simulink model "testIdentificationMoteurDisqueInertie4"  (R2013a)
settings: Solver=ode45  StartTime=0  StopTime=1  FixedStep=1e-3  MaxStep=SimParam2.Te  RelTol=1e-4  AbsTol=1e-4
PreLoadFcn:
  | warning('off','sm:sli:setup:compile:LocalSolverNotSupported')
model workspace (MAT data in the model file):
  handle : class17 (value not decoded)
  handle : class17 (value not decoded)
undefined symbols (not defined in the file or in its folder): SimParam2

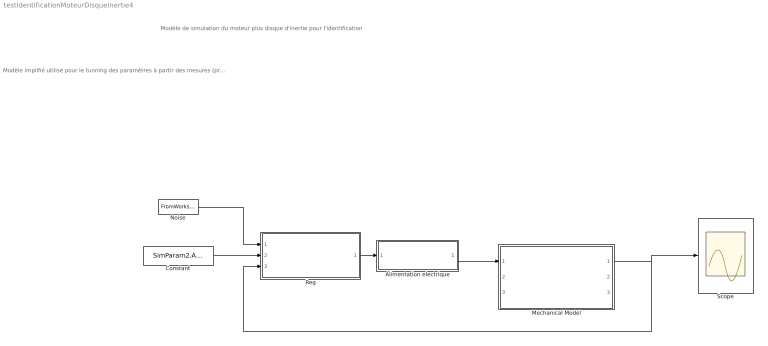
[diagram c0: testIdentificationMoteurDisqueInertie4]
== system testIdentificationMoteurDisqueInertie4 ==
  note: Modèle de simulation du moteur plus disque d'inertie pour l'identification
  note: Modèle implifié utilisé pour le tunning des paramètres à partir des mesures (prbs) effectuée sur le robot (Idem testIdentificationMoteur mais avec un élèment flexible dans le moteur) - Régulateur PID simple avec quantification codeur - Alimentation éléctrique modélisée par une fonction de transfert d'ordre deux avec delais (delais du contrôle) - Méchanique comprennant uniquement un modèle du moteur (inertie + frottement + 1ddl flexible en torsion) + frottement sec - Signaux d'exitation comprennant un bruit blanc et un signal cyclique (PRBS)
  Alimentation electrique : Subsystem
  Constant : Constant  Value=SimParam2.Alpha_c
  Mechanical Model : ModelReference  ModelNameDialog=MotorOnly_sm2.slx  SimulationMode=Normal  ModelReferenceVersion=1.261  CopyOfModelName=MotorOnly_sm2.slx  DefaultDataLogging=on
  Noise : FromWorkspace  VariableName=SimIn  SampleTime=SimParam2.Te  Interpolate=off  OutputAfterFinalValue=Holding final value
  Reg : Subsystem
  Scope : Scope
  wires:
  Noise/1 -> Reg/1(Noise)
  Reg/1(Torque) -> Alimentation electrique/1(Torque_in)
  Constant/1 -> Reg/2(Alpha_c)
  Alimentation electrique/1(Torque_out) -> Mechanical Model/1
  Mechanical Model/1 -> Reg/3(Alpha), Scope/1

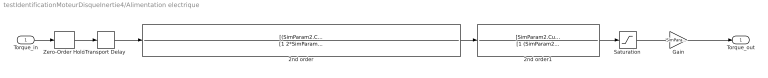
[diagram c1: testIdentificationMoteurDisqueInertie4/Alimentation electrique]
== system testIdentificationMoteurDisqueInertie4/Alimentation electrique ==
  Torque_in : Inport
  2nd order : TransferFcn  Numerator=[(SimParam2.CurrentLoop.f0*2*pi)^2]  Denominator=[1 2*SimParam2.CurrentLoop.Cr*(SimParam2.CurrentLoop.f0*2*pi) (SimParam2.CurrentLoop.f0*2*pi)^2]
  2nd order1 : TransferFcn  Numerator=[SimParam2.CurrentLoop.f1*2*pi]  Denominator=[1 (SimParam2.CurrentLoop.f1*2*pi)]
  Gain : Gain  Gain=SimParam2.Grel
  Saturation : Saturate  UpperLimit=10  LowerLimit=-10
  Transport Delay : TransportDelay  DelayTime=SimParam2.tauElec
  Zero-Order Hold : ZeroOrderHold  SampleTime=SimParam2.TeElec
  Torque_out : Outport
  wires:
  Saturation/1 -> Gain/1
  Torque_in/1 -> Zero-Order Hold/1
  Zero-Order Hold/1 -> Transport Delay/1
  2nd order/1 -> 2nd order1/1
  2nd order1/1 -> Saturation/1
  Gain/1 -> Torque_out/1
  Transport Delay/1 -> 2nd order/1

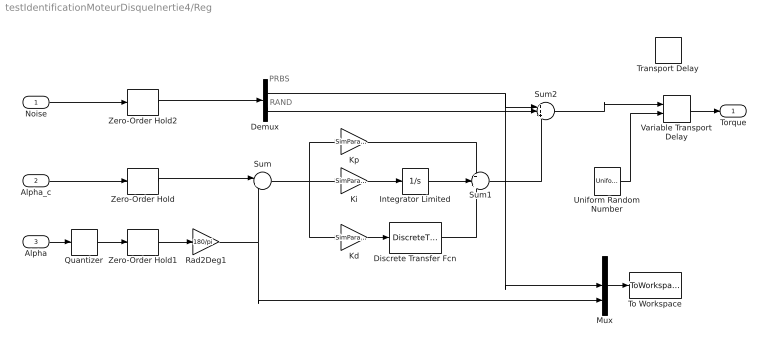
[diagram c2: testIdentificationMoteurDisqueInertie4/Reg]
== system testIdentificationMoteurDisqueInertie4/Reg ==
  note: RAND
  note: PRBS
  Noise : Inport
  Alpha_c : Inport  Port=2
  Alpha : Inport  Port=3
  Demux : Demux  Outputs=2
  Discrete Transfer Fcn : DiscreteTransferFcn  Numerator=[1 0 -1]  Denominator=[2 0 0]
  Integrator Limited : Integrator  LimitOutput=on  UpperSaturationLimit=1  LowerSaturationLimit=-1
  Kd : Gain  Gain=SimParam2.Control.Kd/SimParam2.Te
  Ki : Gain  Gain=SimParam2.Control.Ki*SimParam2.Te
  Kp : Gain  Gain=SimParam2.Control.Kp
  Mux : Mux  Inputs=3
  Quantizer : Quantizer  QuantizationInterval=SimParam2.CoderResol
  Rad2Deg1 : Gain  Gain=180/pi
  Sum : Sum  Inputs=|+-
  Sum1 : Sum  Inputs=+++
  Sum2 : Sum  Inputs=+++
  To Workspace : ToWorkspace  VariableName=simout  SampleTime=SimParam2.Te  SaveFormat=Structure With Time
  Transport Delay : TransportDelay  Commented=on  DelayTime=SimParam2.tauCtr
  Uniform Random Number : UniformRandomNumber  Minimum=SimParam2.tauCtr*0.9  Maximum=SimParam2.tauCtr*1.1  SampleTime=SimParam2.Te
  Variable Transport Delay : VariableTransportDelay  VariableDelayType=Variable transport delay  MaximumDelay=SimParam2.tauCtr*1.2
  Zero-Order Hold : ZeroOrderHold  SampleTime=SimParam2.Te
  Zero-Order Hold1 : ZeroOrderHold  SampleTime=SimParam2.Te
  Zero-Order Hold2 : ZeroOrderHold  SampleTime=SimParam2.Te
  Torque : Outport
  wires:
  Alpha_c/1 -> Zero-Order Hold/1
  Kd/1 -> Discrete Transfer Fcn/1
  Mux/1 -> To Workspace/1
  Zero-Order Hold/1 -> Sum/1
  Alpha/1 -> Quantizer/1
  Quantizer/1 -> Zero-Order Hold1/1
  Noise/1 -> Zero-Order Hold2/1
  Discrete Transfer Fcn/1 -> Sum1/3
  Kp/1 -> Sum1/1
  Sum1/1 -> Sum2/3
  Demux/1 -> Mux/2, Sum2/1
  Ki/1 -> Integrator Limited/1
  Integrator Limited/1 -> Sum1/2
  Sum/1 -> Ki/1, Kp/1, Kd/1
  Zero-Order Hold1/1 -> Rad2Deg1/1
  Rad2Deg1/1 -> Mux/3, Sum/2
  Demux/2 -> Sum2/2
  Zero-Order Hold2/1 -> Demux/1
  Sum2/1 -> Variable Transport Delay/1
  Variable Transport Delay/1 -> Torque/1
  Uniform Random Number/1 -> Variable Transport Delay/2
